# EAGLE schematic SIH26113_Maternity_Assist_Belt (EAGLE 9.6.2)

## Sheet 1 of 7: SHEET 1/7 - POWER ENTRY, CHARGING AND 3V3 REGULATION
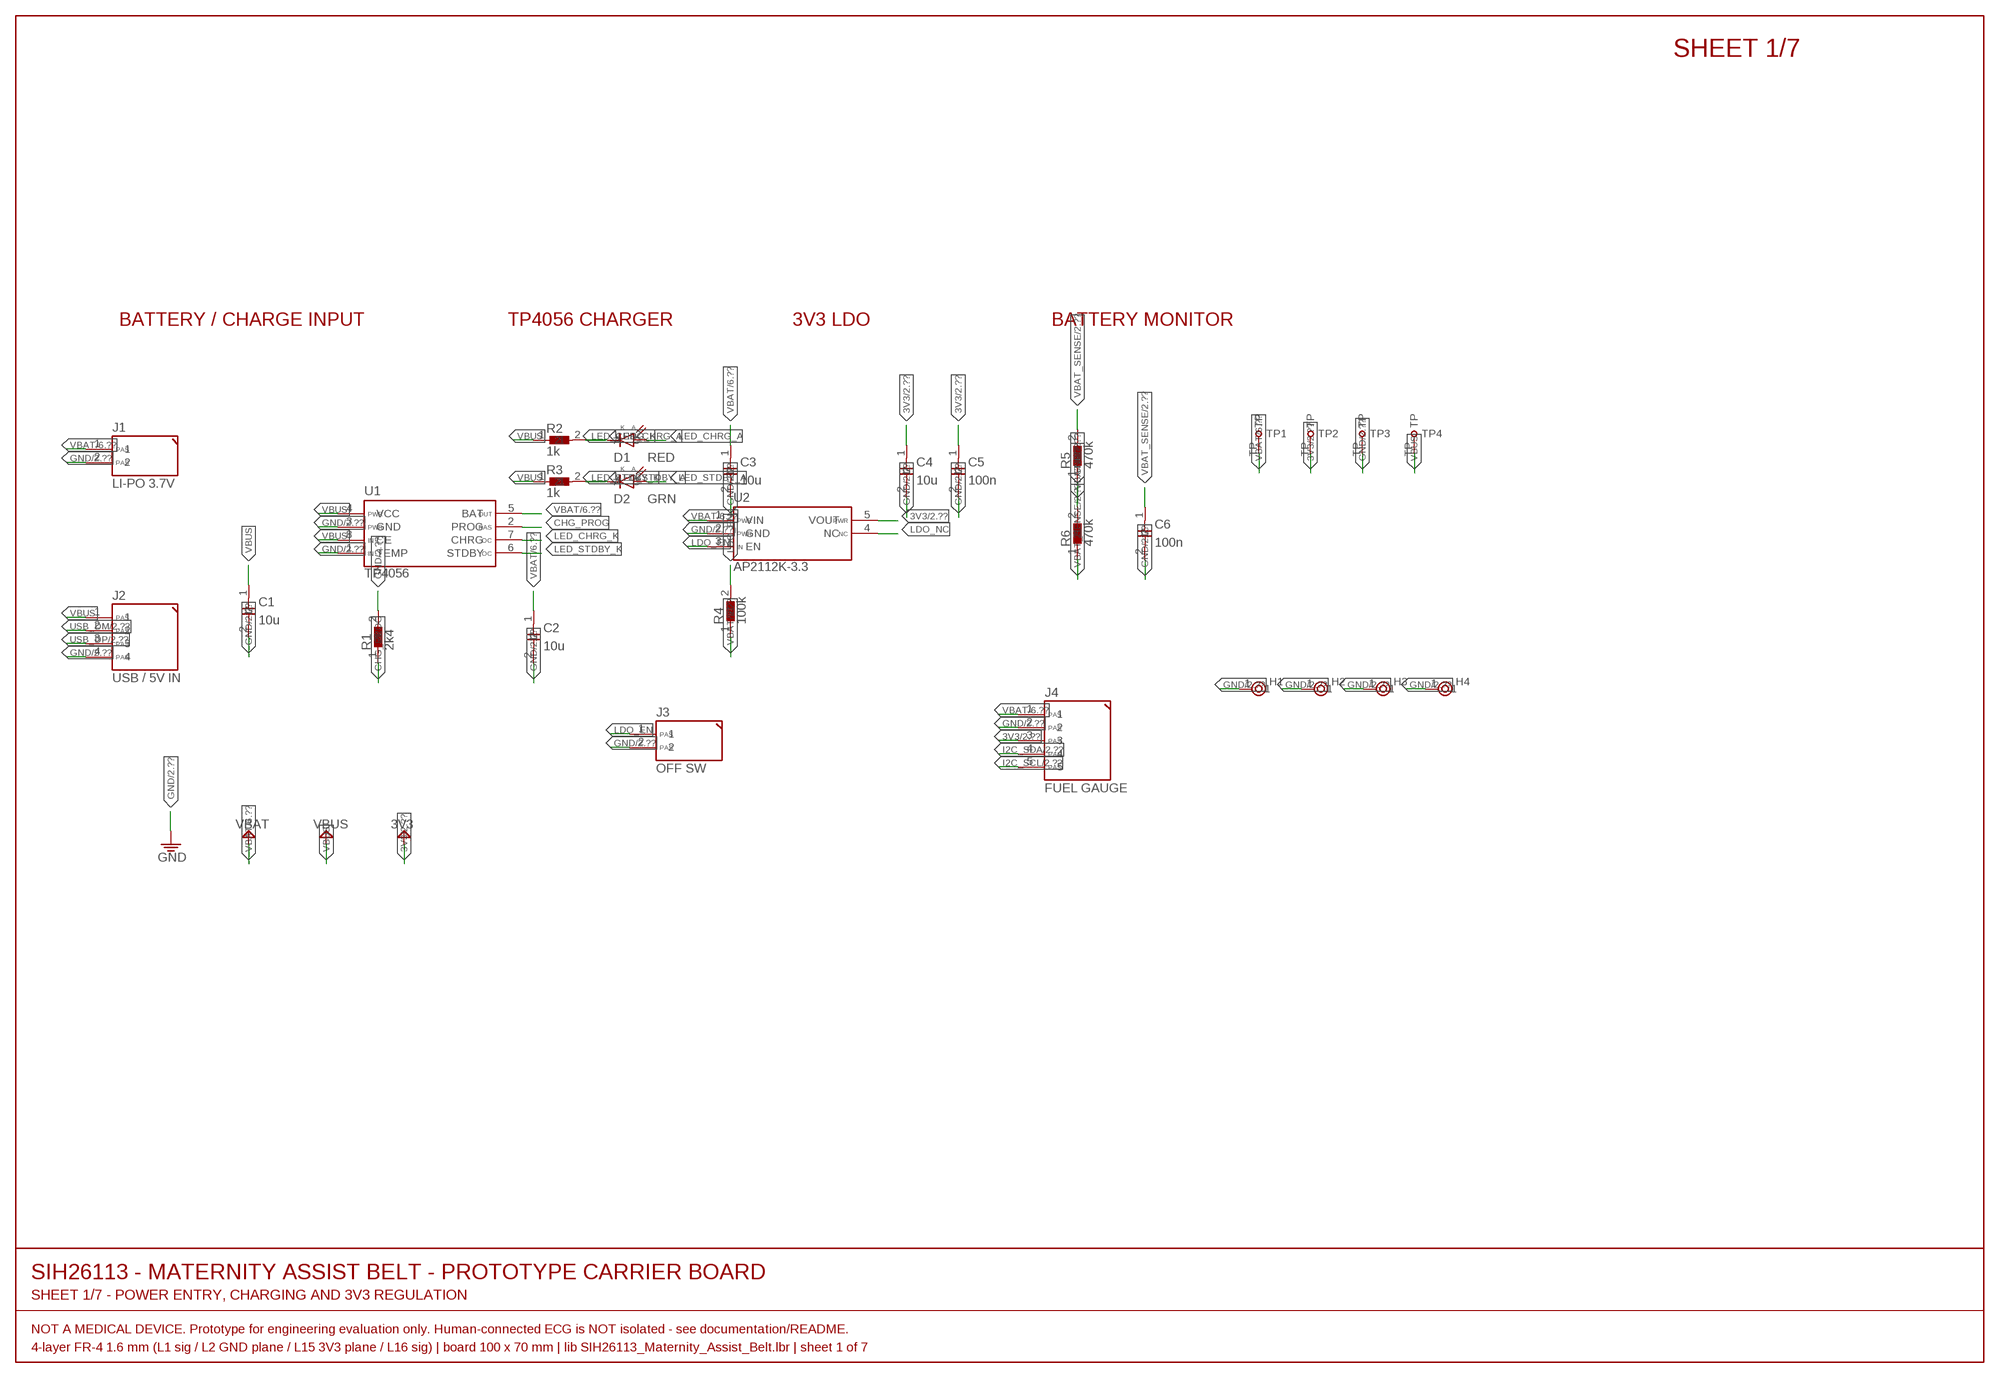
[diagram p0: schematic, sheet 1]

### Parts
C1  10u  C-0805  [C0805]
C2  10u  C-0805  [C0805]
C3  10u  C-0805  [C0805]
C4  10u  C-0805  [C0805]
C5  100n  C-0805  [C0805]
C6  100n  C-0805  [C0805]
D1  RED  LED-0805  [LED0805]
D2  GRN  LED-0805  [LED0805]
H1  M2  MOUNTHOLE-M2  [MOUNT-M2]
H2  M2  MOUNTHOLE-M2  [MOUNT-M2]
H3  M2  MOUNTHOLE-M2  [MOUNT-M2]
H4  M2  MOUNTHOLE-M2  [MOUNT-M2]
J1  LI-PO 3.7V  JST-PH-2  [JST-PH-2]
J2  USB / 5V IN  HDR-1X4  [HDR-1X4]
J3  OFF SW  HDR-1X2  [HDR-1X2]
J4  FUEL GAUGE  HDR-1X5  [HDR-1X5]
R1  2k4  R-0805  [R0805]
R2  1k  R-0805  [R0805]
R3  1k  R-0805  [R0805]
R4  100k  R-0805  [R0805]
R5  470k  R-0805  [R0805]
R6  470k  R-0805  [R0805]
TP1  VBAT  TESTPOINT  [TESTPOINT-1.5]
TP2  3V3  TESTPOINT  [TESTPOINT-1.5]
TP3  GND  TESTPOINT  [TESTPOINT-1.5]
TP4  VBUS  TESTPOINT  [TESTPOINT-1.5]
U1  TP4056  [SOIC-8-N]
U2  AP2112K-3.3  [SOT-23-5]

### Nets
3V3 [power]: C4.1 C5.1 J4.3 TP2.TP U2.5(VOUT) ; also sheet 2,3,4,5,6,7
CHG_PROG: R1.1 U1.2(PROG)
GND [power]: C1.2 C2.2 C3.2 C4.2 C5.2 C6.2 H1.1 H2.1 H3.1 H4.1 J1.2 J2.4 J3.2 J4.2 R1.2 R6.2 TP3.TP U1.1(TEMP) U1.3(GND) U2.2(GND) ; also sheet 2,3,4,5,6,7
I2C_SCL: J4.5 ; also sheet 2,3,7
I2C_SDA: J4.4 ; also sheet 2,3,7
LDO_EN: J3.1 R4.2 U2.3(EN)
LDO_NC: U2.4(NC)
LED_CHRG_A: D1.2(A) R2.2
LED_CHRG_K: D1.1(C) U1.7(CHRG)
LED_STDBY_A: D2.2(A) R3.2
LED_STDBY_K: D2.1(C) U1.6(STDBY)
USB_DM: J2.2 ; also sheet 2
USB_DP: J2.3 ; also sheet 2
VBAT [power]: C2.1 C3.1 J1.1 J4.1 R4.1 R5.1 TP1.TP U1.5(BAT) U2.1(VIN) ; also sheet 6
VBAT_SENSE: C6.1 R5.2 R6.1 ; also sheet 2
VBUS [power]: C1.1 J2.1 R2.1 R3.1 TP4.TP U1.4(VCC) U1.8(CE)

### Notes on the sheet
- SHEET 1/7
- BATTERY / CHARGE INPUT | TP4056 CHARGER | 3V3 LDO | BATTERY MONITOR
- SIH26113 - MATERNITY ASSIST BELT - PROTOTYPE CARRIER BOARD
- SHEET 1/7 - POWER ENTRY, CHARGING AND 3V3 REGULATION
- NOT A MEDICAL DEVICE. Prototype for engineering evaluation only. Human-connected ECG is NOT isolated - see documentation/README.
- 4-layer FR-4 1.6 mm (L1 sig / L2 GND plane / L15 3V3 plane / L16 sig) | board 100 x 70 mm | lib SIH26113_Maternity_Assist_Belt.lbr | sheet 1 of 7

## Sheet 2 of 7: SHEET 2/7 - ESP32-S3 CENTRAL MCU, RESET/BOOT, PROGRAMMING, INDICATORS
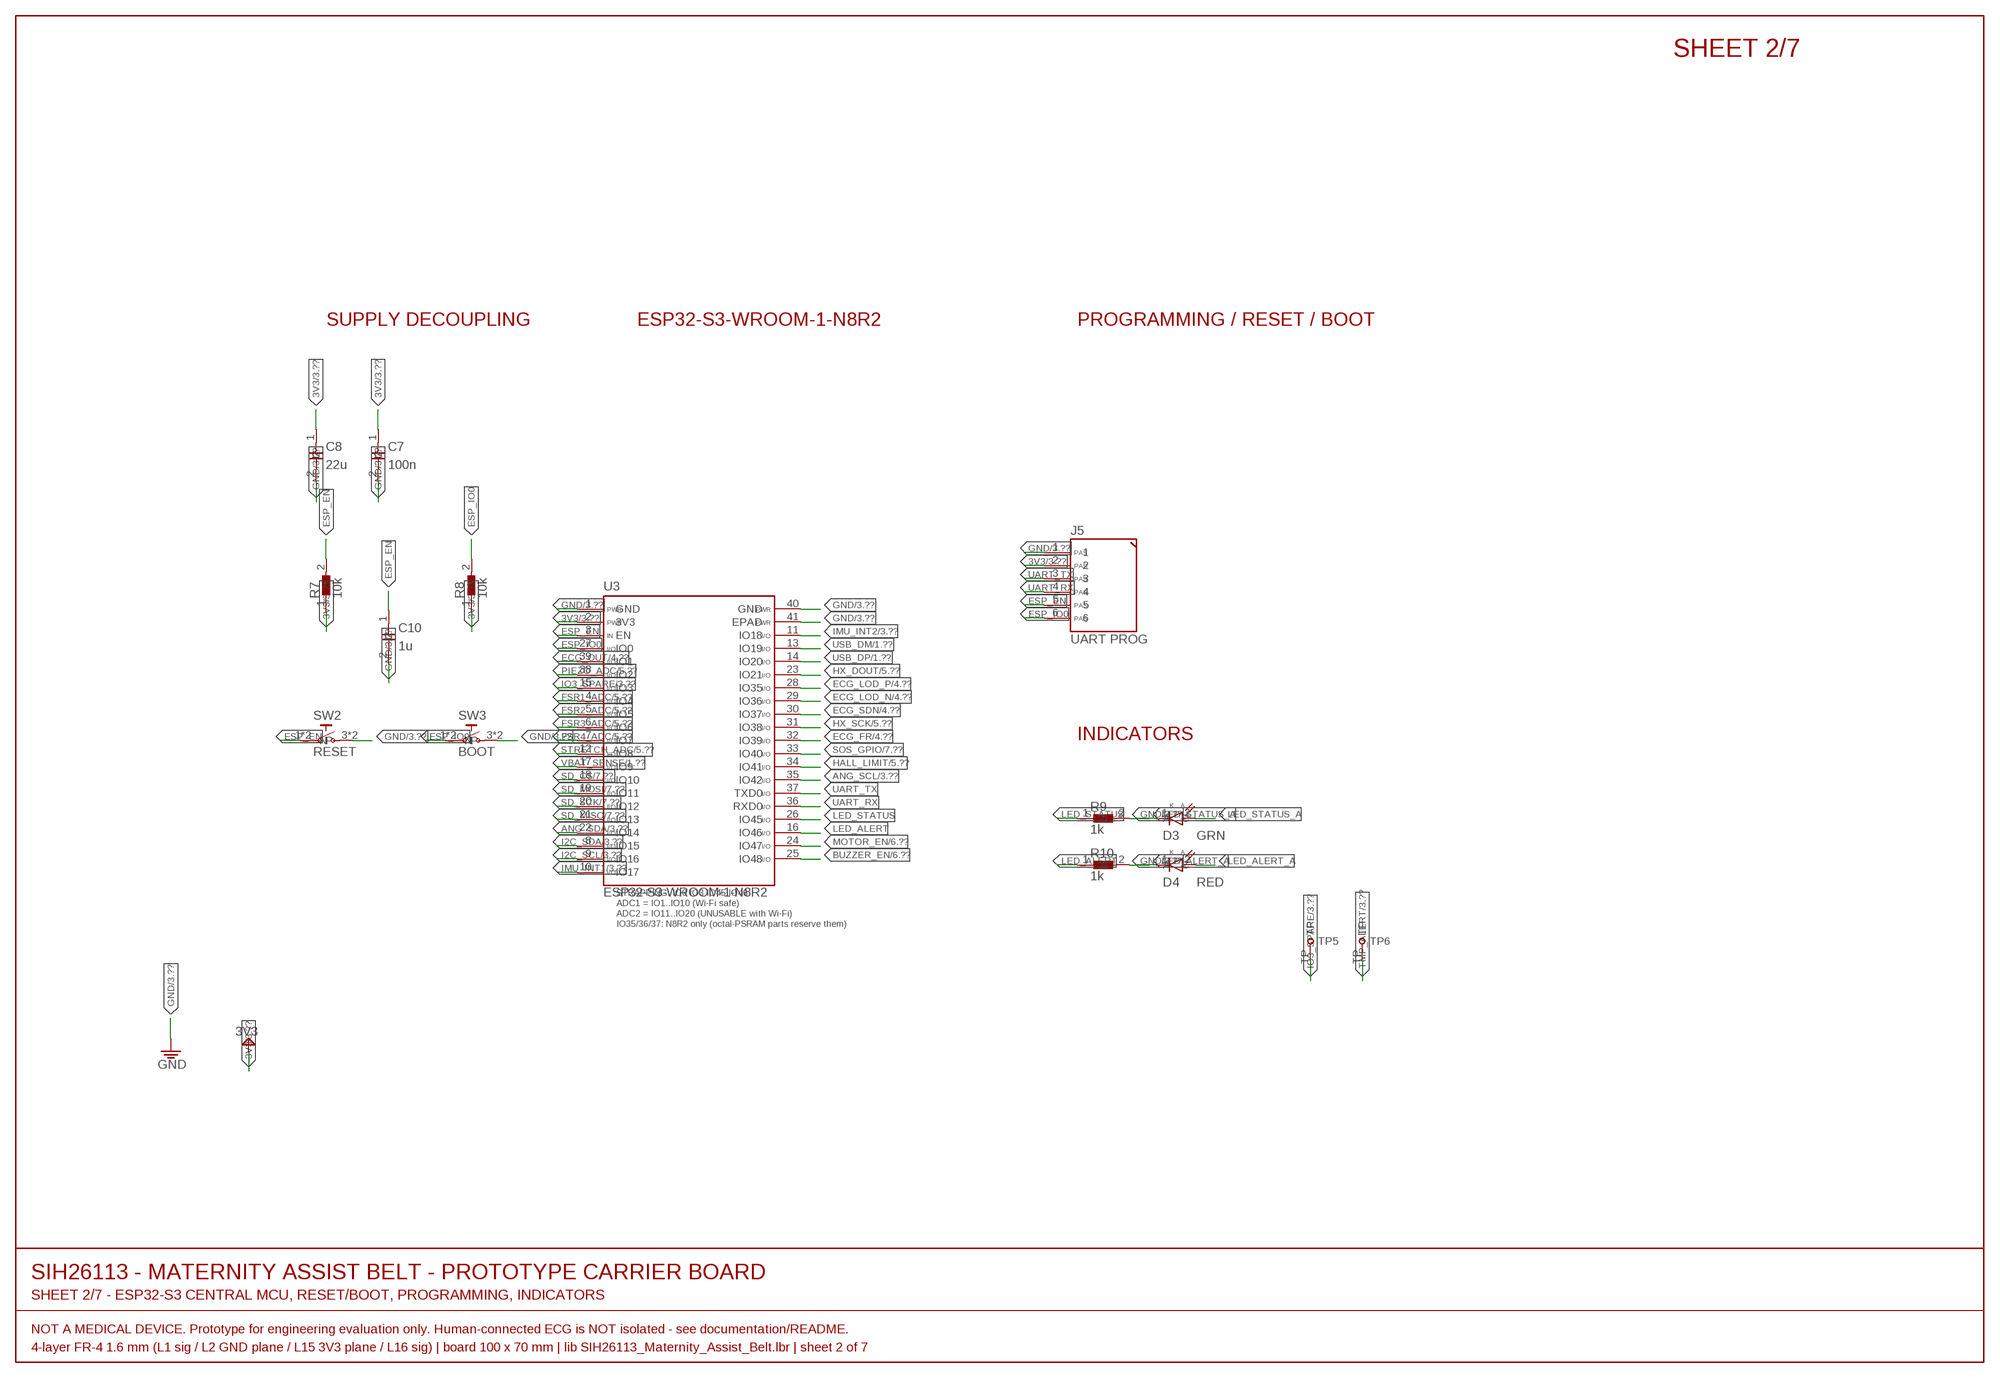
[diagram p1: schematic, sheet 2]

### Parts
C7  100n  C-0805  [C0805]
C8  22u  C-0805  [C0805]
C10  1u  C-0805  [C0805]
D3  GRN  LED-0805  [LED0805]
D4  RED  LED-0805  [LED0805]
J5  UART PROG  HDR-1X6  [HDR-1X6]
R7  10k  R-0805  [R0805]
R8  10k  R-0805  [R0805]
R9  1k  R-0805  [R0805]
R10  1k  R-0805  [R0805]
SW2  RESET  SW-TACT-6MM  [TACT-6X6-THT]
SW3  BOOT  SW-TACT-6MM  [TACT-6X6-THT]
TP5  IO3  TESTPOINT  [TESTPOINT-1.5]
TP6  TMP_ALERT  TESTPOINT  [TESTPOINT-1.5]
U3  ESP32-S3-WROOM-1-N8R2  ESP32-S3-WROOM-1  [ESP32-S3-WROOM-1]

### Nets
3V3 [power]: C7.1 C8.1 J5.2 R7.1 R8.1 U3.2(3V3) ; also sheet 1,3,4,5,6,7
ANG_SCL: U3.35(IO42) ; also sheet 3
ANG_SDA: U3.22(IO14) ; also sheet 3
BUZZER_EN: U3.25(IO48) ; also sheet 6
ECG_FR: U3.32(IO39) ; also sheet 4
ECG_LOD_N: U3.29(IO36) ; also sheet 4
ECG_LOD_P: U3.28(IO35) ; also sheet 4
ECG_OUT [analog_ecg]: U3.39(IO1) ; also sheet 4
ECG_SDN: U3.30(IO37) ; also sheet 4
ESP_EN: C10.1 J5.5 R7.2 SW2.1(P) SW2.2(P) U3.3(EN)
ESP_IO0: J5.6 R8.2 SW3.1(P) SW3.2(P) U3.27(IO0)
FSR1_ADC: U3.4(IO4) ; also sheet 5
FSR2_ADC: U3.5(IO5) ; also sheet 5
FSR3_ADC: U3.6(IO6) ; also sheet 5
FSR4_ADC: U3.7(IO7) ; also sheet 5
GND [power]: C7.2 C8.2 C10.2 D3.1(C) D4.1(C) J5.1 SW2.3(N) SW2.4(N) SW3.3(N) SW3.4(N) U3.1(GND) U3.40(GND) U3.41(EPAD) ; also sheet 1,3,4,5,6,7
HALL_LIMIT: U3.34(IO41) ; also sheet 5
HX_DOUT: U3.23(IO21) ; also sheet 5
HX_SCK: U3.31(IO38) ; also sheet 5
I2C_SCL: U3.9(IO16) ; also sheet 1,3,7
I2C_SDA: U3.8(IO15) ; also sheet 1,3,7
IMU_INT1: U3.10(IO17) ; also sheet 3
IMU_INT2: U3.11(IO18) ; also sheet 3
IO3_SPARE: TP5.TP U3.15(IO3) ; also sheet 3
LED_ALERT: R10.1 U3.16(IO46)
LED_ALERT_A: D4.2(A) R10.2
LED_STATUS: R9.1 U3.26(IO45)
LED_STATUS_A: D3.2(A) R9.2
MOTOR_EN: U3.24(IO47) ; also sheet 6
PIEZO_ADC: U3.38(IO2) ; also sheet 5
SD_CS: U3.18(IO10) ; also sheet 7
SD_MISO: U3.21(IO13) ; also sheet 7
SD_MOSI: U3.19(IO11) ; also sheet 7
SD_SCK: U3.20(IO12) ; also sheet 7
SOS_GPIO: U3.33(IO40) ; also sheet 7
STRETCH_ADC: U3.12(IO8) ; also sheet 5
TMP_ALERT: TP6.TP ; also sheet 3
UART_RX: J5.4 U3.36(RXD0)
UART_TX: J5.3 U3.37(TXD0)
USB_DM: U3.13(IO19) ; also sheet 1
USB_DP: U3.14(IO20) ; also sheet 1
VBAT_SENSE: U3.17(IO9) ; also sheet 1

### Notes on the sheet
- SHEET 2/7
- SUPPLY DECOUPLING | ESP32-S3-WROOM-1-N8R2 | PROGRAMMING / RESET / BOOT
- INDICATORS
- SIH26113 - MATERNITY ASSIST BELT - PROTOTYPE CARRIER BOARD
- SHEET 2/7 - ESP32-S3 CENTRAL MCU, RESET/BOOT, PROGRAMMING, INDICATORS
- NOT A MEDICAL DEVICE. Prototype for engineering evaluation only. Human-connected ECG is NOT isolated - see documentation/README.
- 4-layer FR-4 1.6 mm (L1 sig / L2 GND plane / L15 3V3 plane / L16 sig) | board 100 x 70 mm | lib SIH26113_Maternity_Assist_Belt.lbr | sheet 2 of 7

## Sheet 3 of 7: SHEET 3/7 - I2C SENSORS (TMP117, LSM6DSOX, AS5600) - TWO BUSSES
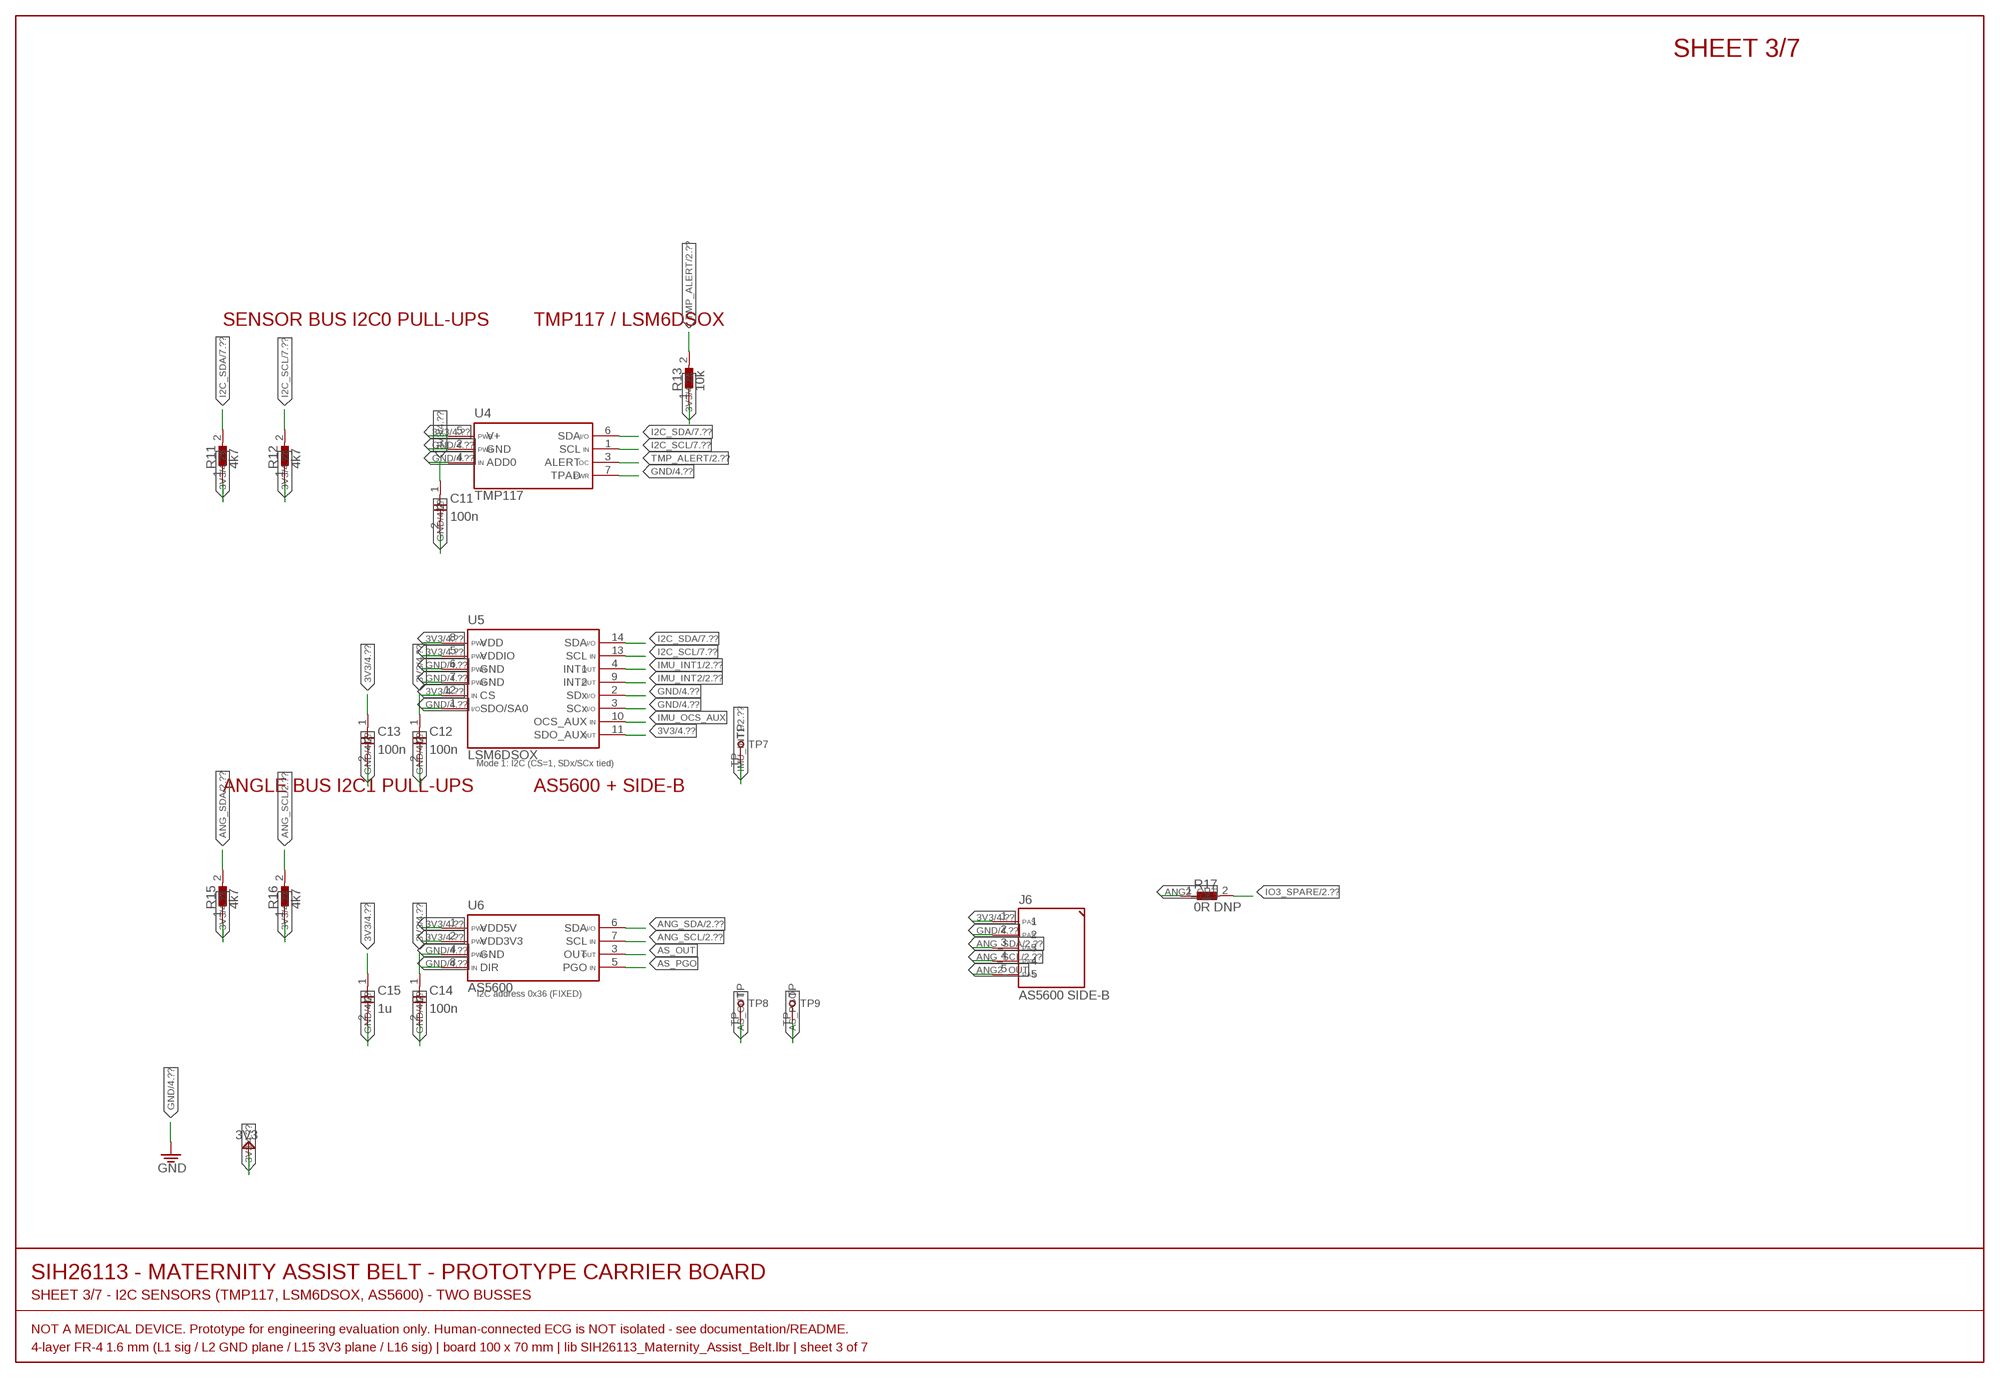
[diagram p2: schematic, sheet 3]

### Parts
C11  100n  C-0805  [C0805]
C12  100n  C-0805  [C0805]
C13  100n  C-0805  [C0805]
C14  100n  C-0805  [C0805]
C15  1u  C-0805  [C0805]
J6  AS5600 SIDE-B  HDR-1X5  [HDR-1X5]
R11  4k7  R-0805  [R0805]
R12  4k7  R-0805  [R0805]
R13  10k  R-0805  [R0805]
R15  4k7  R-0805  [R0805]
R16  4k7  R-0805  [R0805]
R17  0R DNP  R-0805  [R0805]
TP7  IMU_INT1  TESTPOINT  [TESTPOINT-1.5]
TP8  AS_OUT  TESTPOINT  [TESTPOINT-1.5]
TP9  AS_PGO  TESTPOINT  [TESTPOINT-1.5]
U4  TMP117  [WSON-6-DRV0006B]
U5  LSM6DSOX  [LGA-14L-2.5X3.0]
U6  AS5600  [SOIC-8-N]

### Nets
3V3 [power]: C11.1 C12.1 C13.1 C14.1 C15.1 J6.1 R11.1 R12.1 R13.1 R15.1 R16.1 U4.5(V+) U5.5(VDDIO) U5.8(VDD) U5.11(SDO_AUX) U5.12(CS) U6.1(VDD5V) U6.2(VDD3V3) ; also sheet 1,2,4,5,6,7
ANG2_OUT: J6.5 R17.1
ANG_SCL: J6.4 R16.2 U6.7(SCL) ; also sheet 2
ANG_SDA: J6.3 R15.2 U6.6(SDA) ; also sheet 2
AS_OUT: TP8.TP U6.3(OUT)
AS_PGO: TP9.TP U6.5(PGO)
GND [power]: C11.2 C12.2 C13.2 C14.2 C15.2 J6.2 U4.2(GND) U4.4(ADD0) U4.7(TPAD) U5.1(SDO/SA0) U5.2(SDx) U5.3(SCx) U5.6(GND) U5.7(GND) U6.4(GND) U6.8(DIR) ; also sheet 1,2,4,5,6,7
I2C_SCL: R12.2 U4.1(SCL) U5.13(SCL) ; also sheet 1,2,7
I2C_SDA: R11.2 U4.6(SDA) U5.14(SDA) ; also sheet 1,2,7
IMU_INT1: TP7.TP U5.4(INT1) ; also sheet 2
IMU_INT2: U5.9(INT2) ; also sheet 2
IMU_OCS_AUX: U5.10(OCS_AUX)
IO3_SPARE: R17.2 ; also sheet 2
TMP_ALERT: R13.2 U4.3(ALERT) ; also sheet 2

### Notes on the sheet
- SHEET 3/7
- SENSOR BUS I2C0 PULL-UPS | TMP117 / LSM6DSOX
- ANGLE BUS I2C1 PULL-UPS | AS5600 + SIDE-B
- SIH26113 - MATERNITY ASSIST BELT - PROTOTYPE CARRIER BOARD
- SHEET 3/7 - I2C SENSORS (TMP117, LSM6DSOX, AS5600) - TWO BUSSES
- NOT A MEDICAL DEVICE. Prototype for engineering evaluation only. Human-connected ECG is NOT isolated - see documentation/README.
- 4-layer FR-4 1.6 mm (L1 sig / L2 GND plane / L15 3V3 plane / L16 sig) | board 100 x 70 mm | lib SIH26113_Maternity_Assist_Belt.lbr | sheet 3 of 7

## Sheet 4 of 7: SHEET 4/7 - ECG ANALOG FRONT END (AD8232)
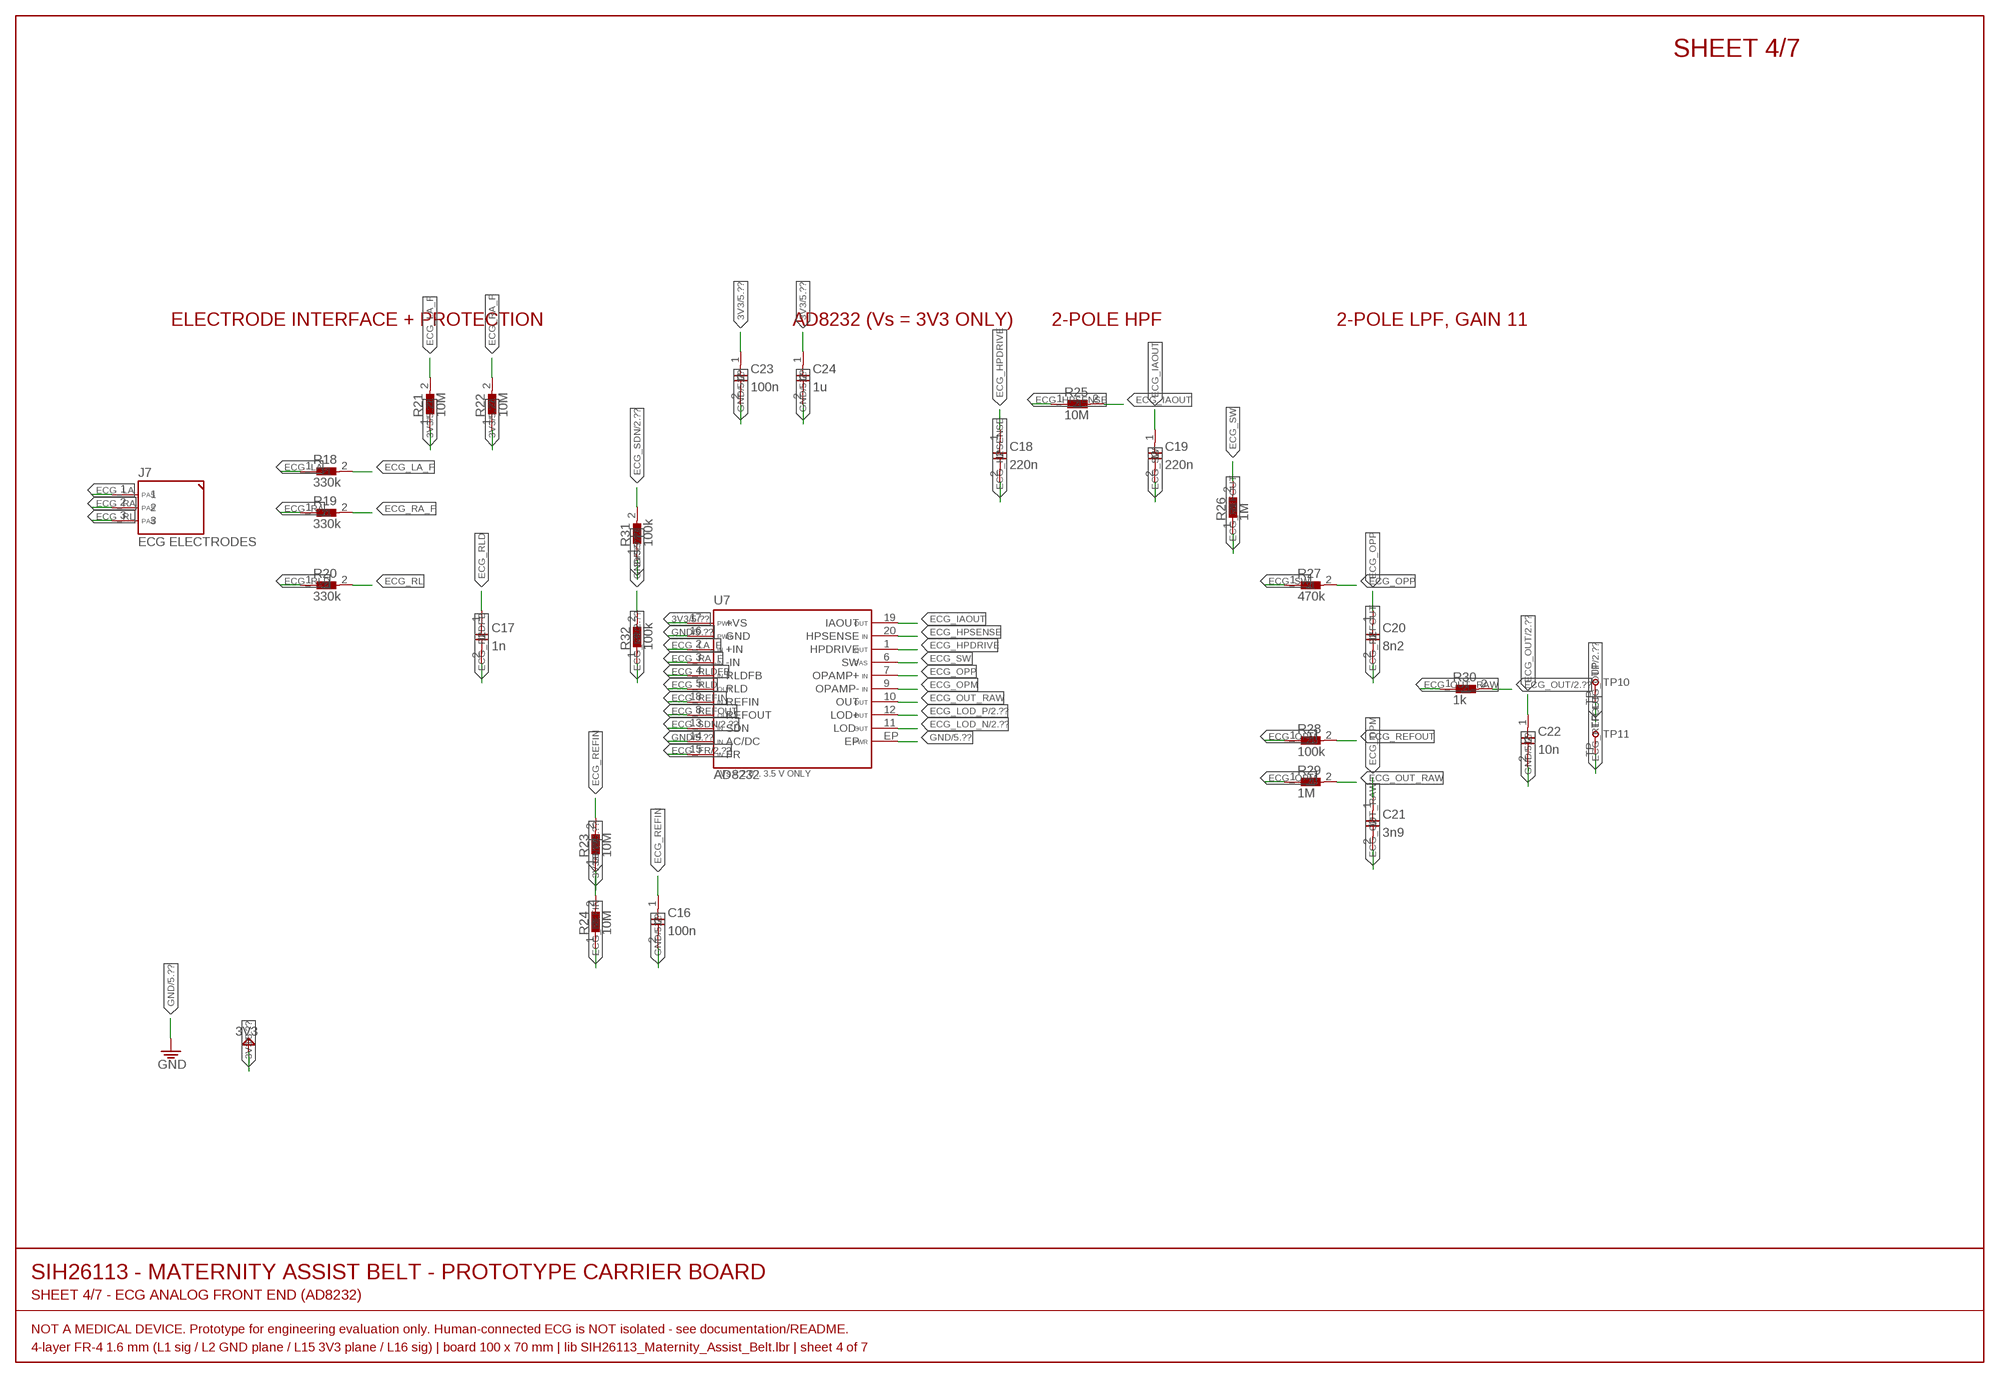
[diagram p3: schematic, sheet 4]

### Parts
C16  100n  C-0805  [C0805]
C17  1n  C-0805  [C0805]
C18  220n  C-0805  [C0805]
C19  220n  C-0805  [C0805]
C20  8n2  C-0805  [C0805]
C21  3n9  C-0805  [C0805]
C22  10n  C-0805  [C0805]
C23  100n  C-0805  [C0805]
C24  1u  C-0805  [C0805]
J7  ECG ELECTRODES  HDR-1X3  [HDR-1X3]
R18  330k  R-0805  [R0805]
R19  330k  R-0805  [R0805]
R20  330k  R-0805  [R0805]
R21  10M  R-0805  [R0805]
R22  10M  R-0805  [R0805]
R23  10M  R-0805  [R0805]
R24  10M  R-0805  [R0805]
R25  10M  R-0805  [R0805]
R26  1M  R-0805  [R0805]
R27  470k  R-0805  [R0805]
R28  100k  R-0805  [R0805]
R29  1M  R-0805  [R0805]
R30  1k  R-0805  [R0805]
R31  100k  R-0805  [R0805]
R32  100k  R-0805  [R0805]
TP10  ECG_OUT  TESTPOINT  [TESTPOINT-1.5]
TP11  ECG_REF  TESTPOINT  [TESTPOINT-1.5]
U7  AD8232  [LFCSP-20-4X4-P050]

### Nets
3V3 [power]: C23.1 C24.1 R21.1 R22.1 R23.1 R31.1 U7.17(+VS) ; also sheet 1,2,3,5,6,7
ECG_FR: R32.1 U7.15(FR) ; also sheet 2
ECG_HPDRIVE: C18.1 U7.1(HPDRIVE)
ECG_HPSENSE [analog_ecg]: C18.2 R25.1 U7.20(HPSENSE)
ECG_IAOUT [analog_ecg]: C19.1 R25.2 U7.19(IAOUT)
ECG_LA [analog_ecg]: J7.1 R18.1
ECG_LA_F [analog_ecg]: R18.2 R21.2 U7.2(+IN)
ECG_LOD_N: U7.11(LOD-) ; also sheet 2
ECG_LOD_P: U7.12(LOD+) ; also sheet 2
ECG_OPM [analog_ecg]: C21.1 R28.1 R29.1 U7.9(OPAMP-)
ECG_OPP [analog_ecg]: C20.1 R27.2 U7.7(OPAMP+)
ECG_OUT [analog_ecg]: C22.1 R30.2 TP10.TP ; also sheet 2
ECG_OUT_RAW [analog_ecg]: C21.2 R29.2 R30.1 U7.10(OUT)
ECG_RA [analog_ecg]: J7.2 R19.1
ECG_RA_F [analog_ecg]: R19.2 R22.2 U7.3(-IN)
ECG_REFIN [analog_ecg]: C16.1 R23.2 R24.1 U7.18(REFIN)
ECG_REFOUT [analog_ecg]: C20.2 R26.1 R28.2 TP11.TP U7.8(REFOUT)
ECG_RL [analog_ecg]: J7.3 R20.2
ECG_RLD [analog_ecg]: C17.1 R20.1 U7.5(RLD)
ECG_RLDFB: C17.2 U7.4(RLDFB)
ECG_SDN: R31.2 U7.13(SDN) ; also sheet 2
ECG_SW [analog_ecg]: C19.2 R26.2 R27.1 U7.6(SW)
GND [power]: C16.2 C22.2 C23.2 C24.2 R24.2 R32.2 U7.14(AC/DC) U7.16(GND) U7.EP ; also sheet 1,2,3,5,6,7

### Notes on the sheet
- SHEET 4/7
- ELECTRODE INTERFACE + PROTECTION | AD8232 (Vs = 3V3 ONLY) | 2-POLE HPF | 2-POLE LPF, GAIN 11
- SIH26113 - MATERNITY ASSIST BELT - PROTOTYPE CARRIER BOARD
- SHEET 4/7 - ECG ANALOG FRONT END (AD8232)
- NOT A MEDICAL DEVICE. Prototype for engineering evaluation only. Human-connected ECG is NOT isolated - see documentation/README.
- 4-layer FR-4 1.6 mm (L1 sig / L2 GND plane / L15 3V3 plane / L16 sig) | board 100 x 70 mm | lib SIH26113_Maternity_Assist_Belt.lbr | sheet 4 of 7

## Sheet 5 of 7: SHEET 5/7 - MECHANICAL SENSING (LOAD CELL, FSR, STRETCH, PIEZO, HALL)
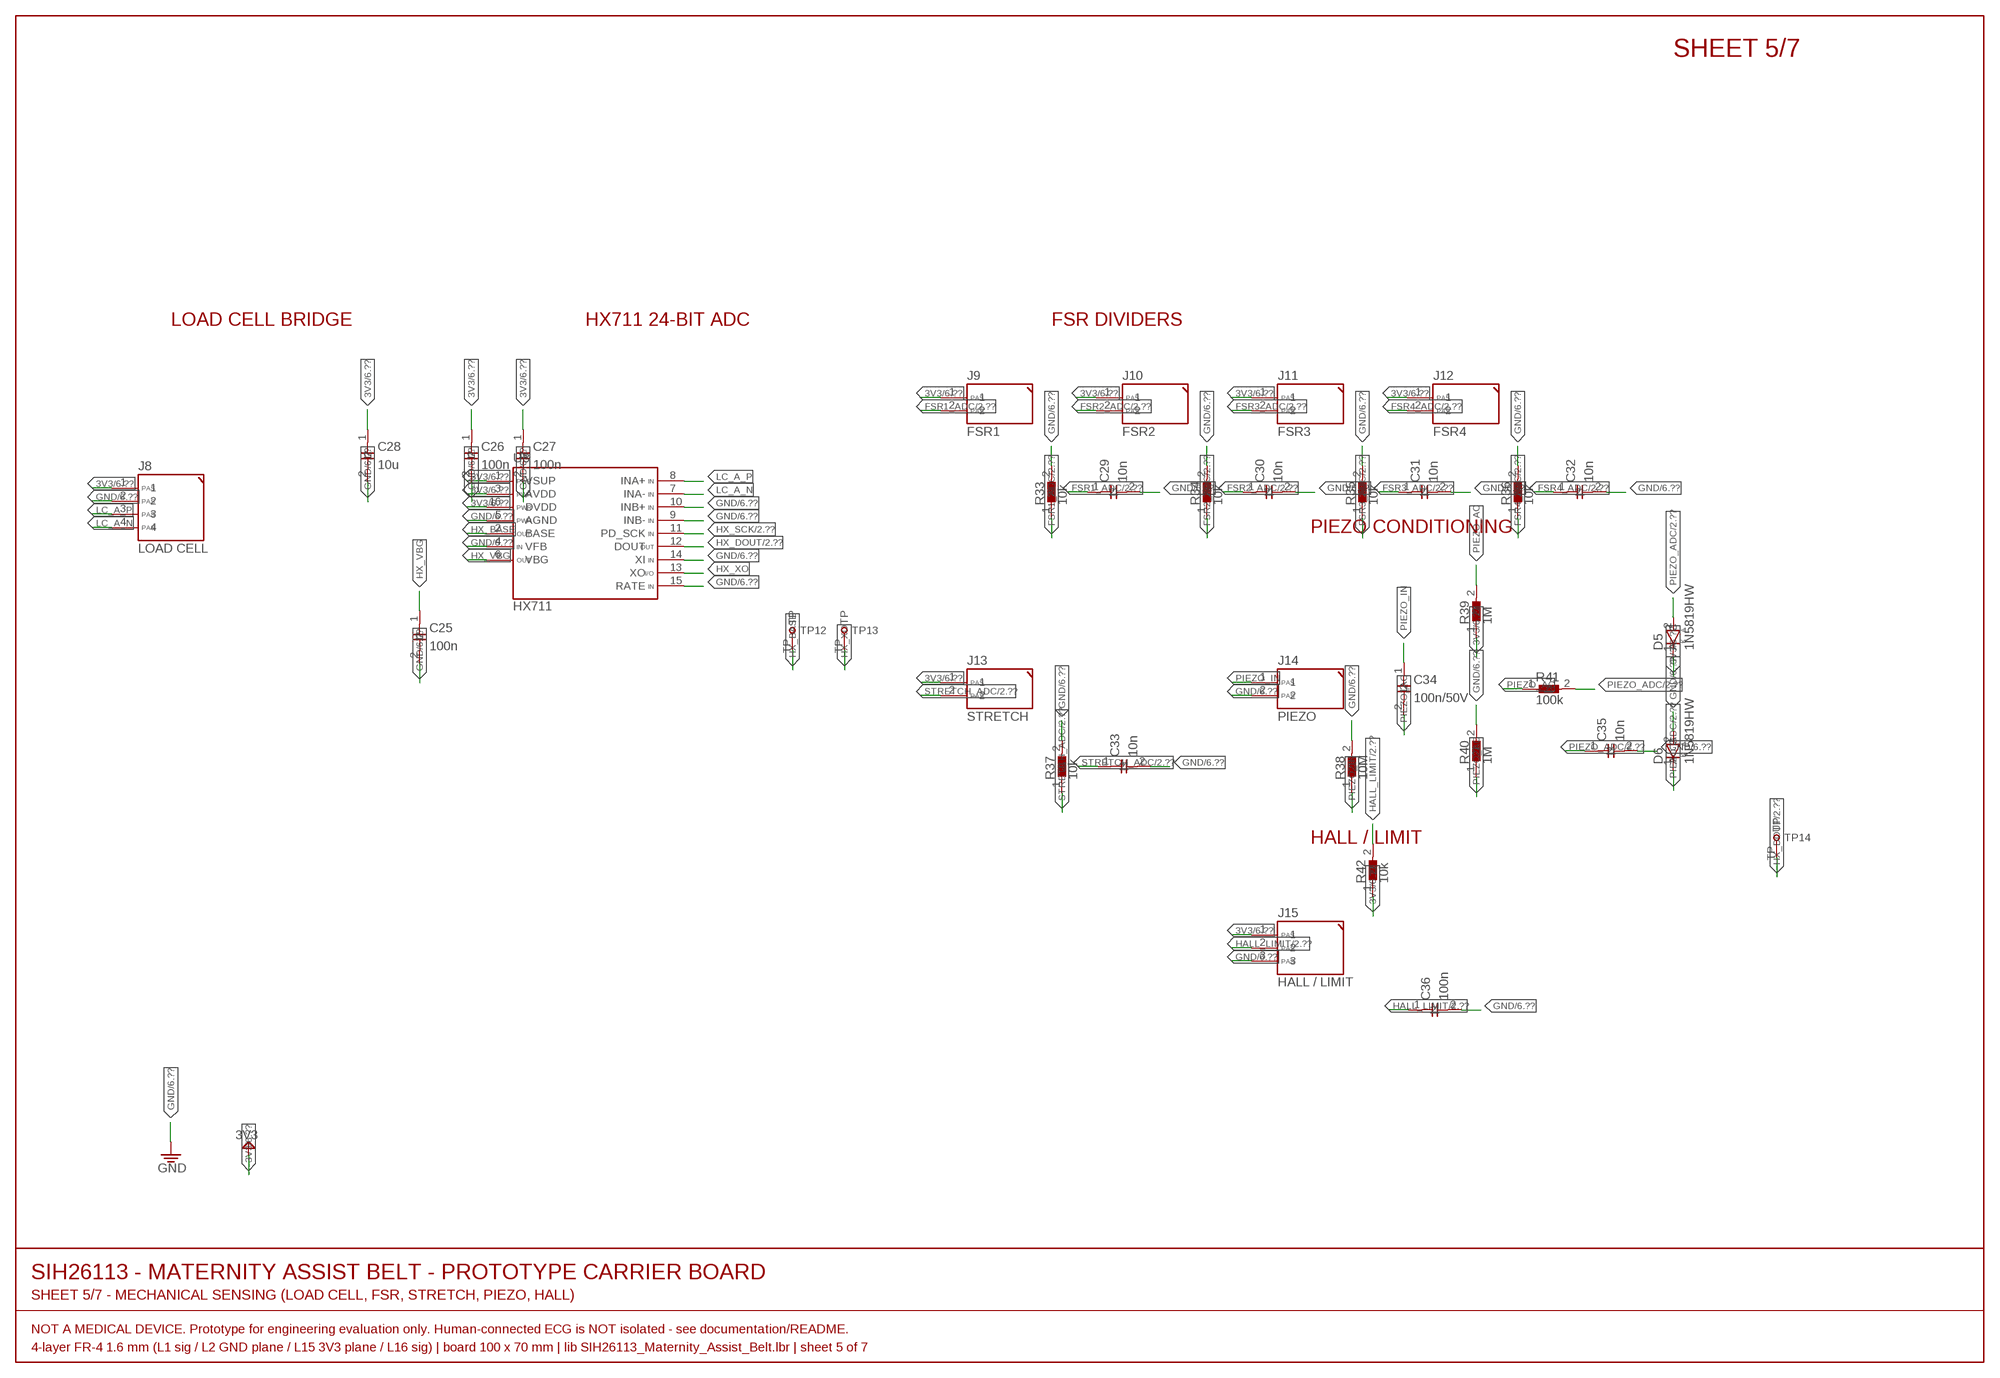
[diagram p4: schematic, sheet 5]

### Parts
C25  100n  C-0805  [C0805]
C26  100n  C-0805  [C0805]
C27  100n  C-0805  [C0805]
C28  10u  C-0805  [C0805]
C29  10n  C-0805  [C0805]
C30  10n  C-0805  [C0805]
C31  10n  C-0805  [C0805]
C32  10n  C-0805  [C0805]
C33  10n  C-0805  [C0805]
C34  100n/50V  C-0805  [C0805]
C35  10n  C-0805  [C0805]
C36  100n  C-0805  [C0805]
D5  1N5819HW  DIODE-SOD123  [SOD-123]
D6  1N5819HW  DIODE-SOD123  [SOD-123]
J8  LOAD CELL  JST-PH-4  [JST-PH-4]
J9  FSR1  HDR-1X2  [HDR-1X2]
J10  FSR2  HDR-1X2  [HDR-1X2]
J11  FSR3  HDR-1X2  [HDR-1X2]
J12  FSR4  HDR-1X2  [HDR-1X2]
J13  STRETCH  HDR-1X2  [HDR-1X2]
J14  PIEZO  HDR-1X2  [HDR-1X2]
J15  HALL / LIMIT  HDR-1X3  [HDR-1X3]
R33  10k  R-0805  [R0805]
R34  10k  R-0805  [R0805]
R35  10k  R-0805  [R0805]
R36  10k  R-0805  [R0805]
R37  10k  R-0805  [R0805]
R38  10M  R-0805  [R0805]
R39  1M  R-0805  [R0805]
R40  1M  R-0805  [R0805]
R41  100k  R-0805  [R0805]
R42  10k  R-0805  [R0805]
TP12  HX_BASE  TESTPOINT  [TESTPOINT-1.5]
TP13  HX_XO  TESTPOINT  [TESTPOINT-1.5]
TP14  HX_DOUT  TESTPOINT  [TESTPOINT-1.5]
U8  HX711  [SOP-16-N]

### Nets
3V3 [power]: C26.1 C27.1 C28.1 D5.1(C) J8.1 J9.1 J10.1 J11.1 J12.1 J13.1 J15.1 R39.1 R42.1 U8.1(VSUP) U8.3(AVDD) U8.16(DVDD) ; also sheet 1,2,3,4,6,7
FSR1_ADC: C29.1 J9.2 R33.1 ; also sheet 2
FSR2_ADC: C30.1 J10.2 R34.1 ; also sheet 2
FSR3_ADC: C31.1 J11.2 R35.1 ; also sheet 2
FSR4_ADC: C32.1 J12.2 R36.1 ; also sheet 2
GND [power]: C25.2 C26.2 C27.2 C28.2 C29.2 C30.2 C31.2 C32.2 C33.2 C35.2 C36.2 D6.2(A) J8.2 J14.2 J15.3 R33.2 R34.2 R35.2 R36.2 R37.2 R38.2 R40.2 U8.4(VFB) U8.5(AGND) U8.9(INB-) U8.10(INB+) U8.14(XI) U8.15(RATE) ; also sheet 1,2,3,4,6,7
HALL_LIMIT: C36.1 J15.2 R42.2 ; also sheet 2
HX_BASE: TP12.TP U8.2(BASE)
HX_DOUT: TP14.TP U8.12(DOUT) ; also sheet 2
HX_SCK: U8.11(PD_SCK) ; also sheet 2
HX_VBG: C25.1 U8.6(VBG)
HX_XO: TP13.TP U8.13(XO)
LC_A_N: J8.4 U8.7(INA-)
LC_A_P: J8.3 U8.8(INA+)
PIEZO_AC: C34.2 R39.2 R40.1 R41.1
PIEZO_ADC: C35.1 D5.2(A) D6.1(C) R41.2 ; also sheet 2
PIEZO_IN: C34.1 J14.1 R38.1
STRETCH_ADC: C33.1 J13.2 R37.1 ; also sheet 2

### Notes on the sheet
- SHEET 5/7
- LOAD CELL BRIDGE | HX711 24-BIT ADC | FSR DIVIDERS
- PIEZO CONDITIONING
- HALL / LIMIT
- SIH26113 - MATERNITY ASSIST BELT - PROTOTYPE CARRIER BOARD
- SHEET 5/7 - MECHANICAL SENSING (LOAD CELL, FSR, STRETCH, PIEZO, HALL)
- NOT A MEDICAL DEVICE. Prototype for engineering evaluation only. Human-connected ECG is NOT isolated - see documentation/README.
- 4-layer FR-4 1.6 mm (L1 sig / L2 GND plane / L15 3V3 plane / L16 sig) | board 100 x 70 mm | lib SIH26113_Maternity_Assist_Belt.lbr | sheet 5 of 7

## Sheet 6 of 7: SHEET 6/7 - FET-DRIVEN ALERTS (VIBRATION MOTOR, BUZZER)
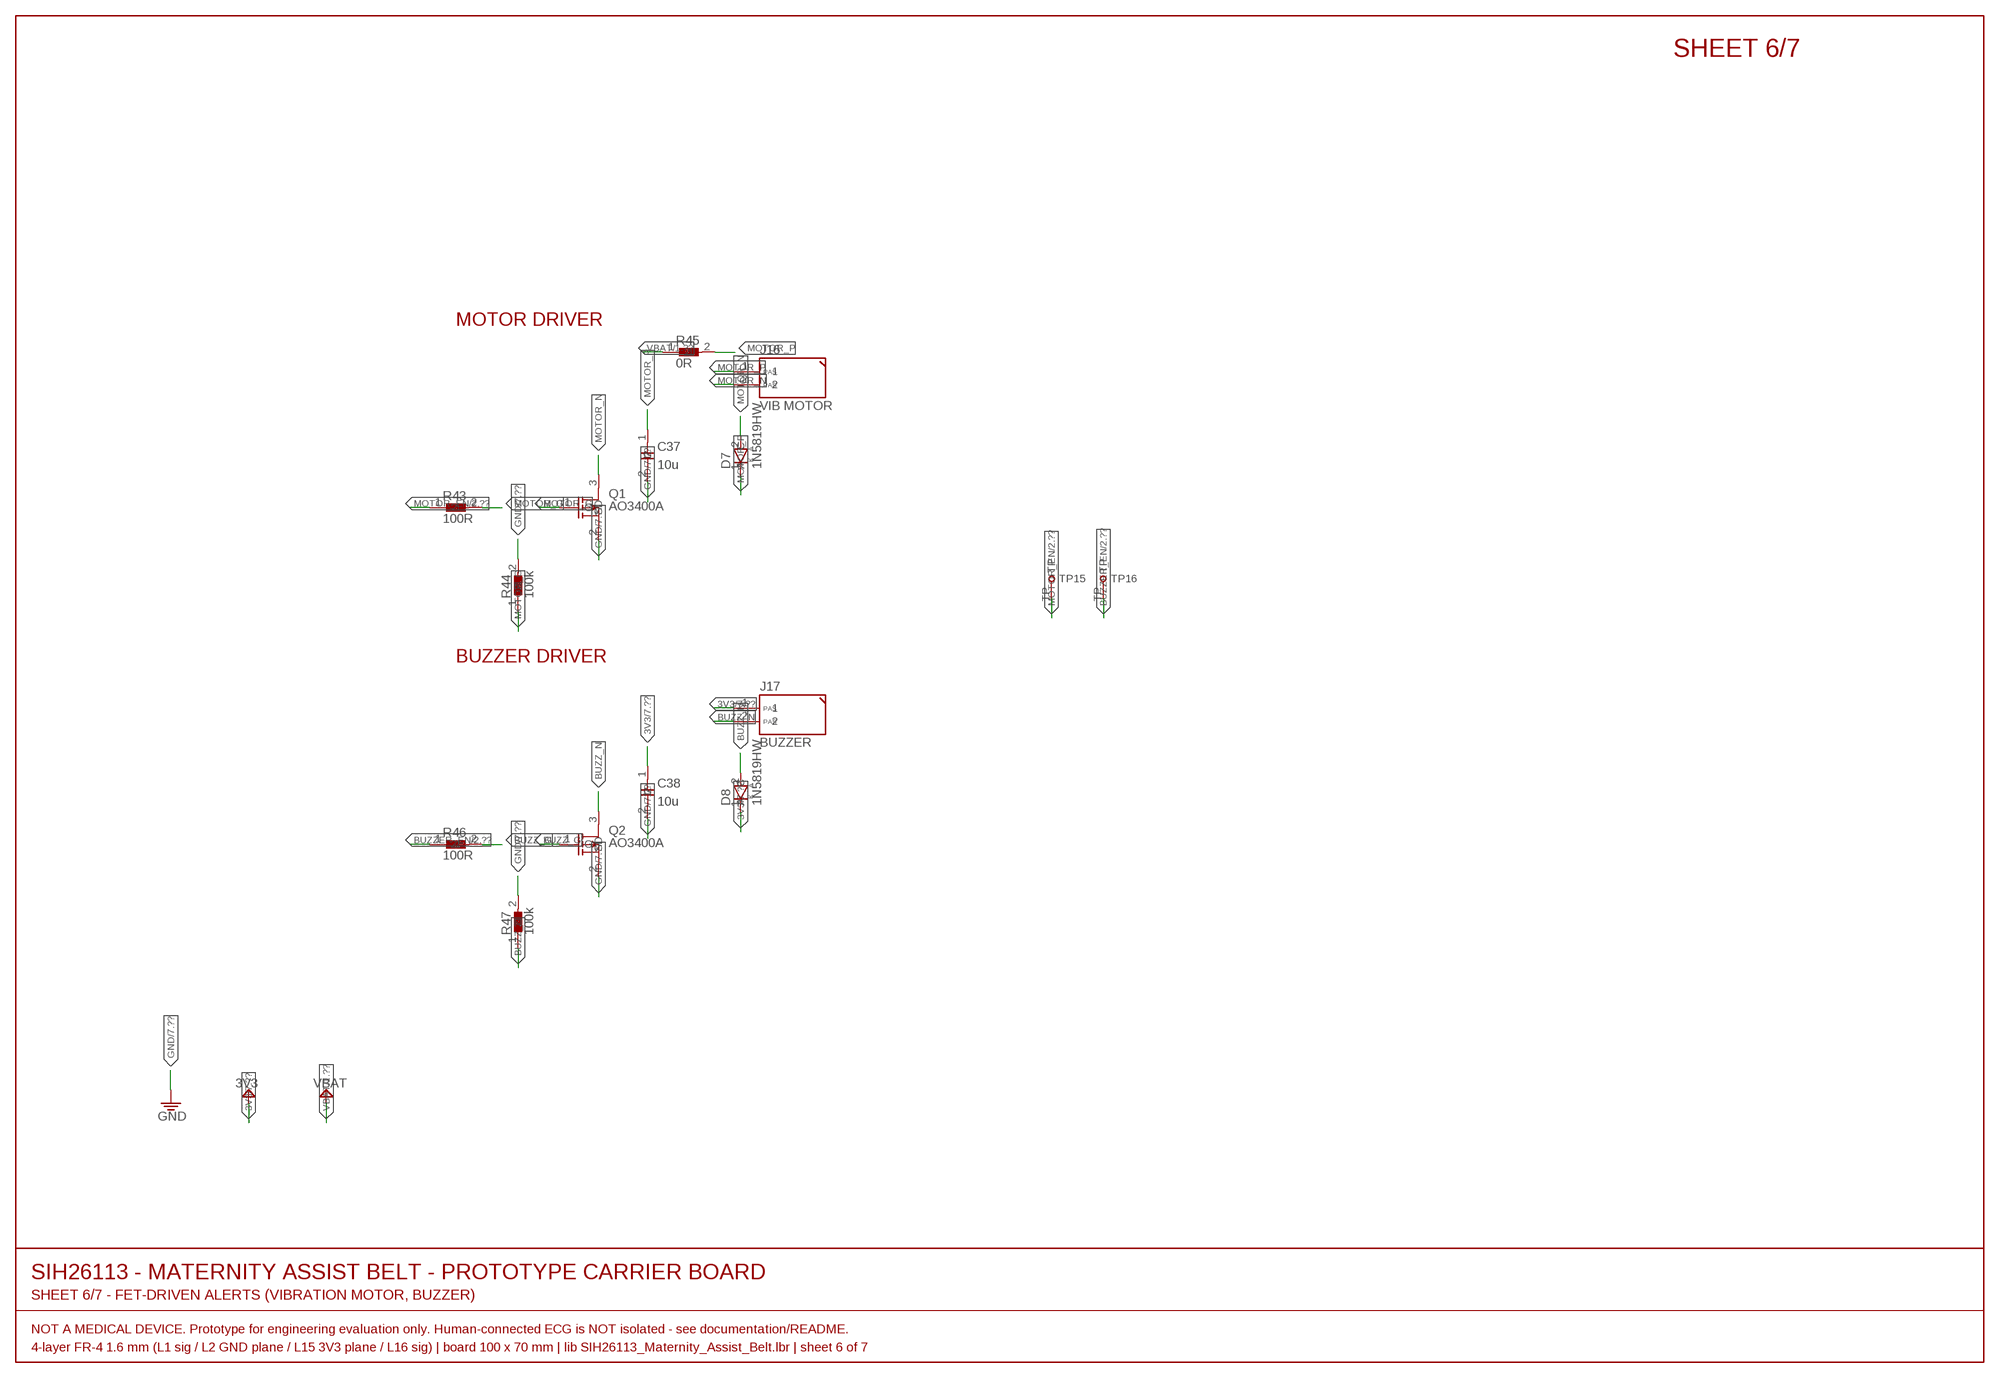
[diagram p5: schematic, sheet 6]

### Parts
C37  10u  C-0805  [C0805]
C38  10u  C-0805  [C0805]
D7  1N5819HW  DIODE-SOD123  [SOD-123]
D8  1N5819HW  DIODE-SOD123  [SOD-123]
J16  VIB MOTOR  HDR-1X2  [HDR-1X2]
J17  BUZZER  HDR-1X2  [HDR-1X2]
Q1  AO3400A  NMOS-SOT23  [SOT-23-3]
Q2  AO3400A  NMOS-SOT23  [SOT-23-3]
R43  100R  R-0805  [R0805]
R44  100k  R-0805  [R0805]
R45  0R  R-0805  [R0805]
R46  100R  R-0805  [R0805]
R47  100k  R-0805  [R0805]
TP15  MOTOR_EN  TESTPOINT  [TESTPOINT-1.5]
TP16  BUZZER_EN  TESTPOINT  [TESTPOINT-1.5]

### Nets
3V3 [power]: C38.1 D8.1(C) J17.1 ; also sheet 1,2,3,4,5,7
BUZZ_G: Q2.1(G) R46.2 R47.1
BUZZ_N: D8.2(A) J17.2 Q2.3(D)
BUZZER_EN: R46.1 TP16.TP ; also sheet 2
GND [power]: C37.2 C38.2 Q1.2(S) Q2.2(S) R44.2 R47.2 ; also sheet 1,2,3,4,5,7
MOTOR_EN: R43.1 TP15.TP ; also sheet 2
MOTOR_G: Q1.1(G) R43.2 R44.1
MOTOR_N [motor]: D7.2(A) J16.2 Q1.3(D)
MOTOR_P [motor]: C37.1 D7.1(C) J16.1 R45.2
VBAT [power]: R45.1 ; also sheet 1

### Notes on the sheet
- SHEET 6/7
- MOTOR DRIVER
- BUZZER DRIVER
- SIH26113 - MATERNITY ASSIST BELT - PROTOTYPE CARRIER BOARD
- SHEET 6/7 - FET-DRIVEN ALERTS (VIBRATION MOTOR, BUZZER)
- NOT A MEDICAL DEVICE. Prototype for engineering evaluation only. Human-connected ECG is NOT isolated - see documentation/README.
- 4-layer FR-4 1.6 mm (L1 sig / L2 GND plane / L15 3V3 plane / L16 sig) | board 100 x 70 mm | lib SIH26113_Maternity_Assist_Belt.lbr | sheet 6 of 7

## Sheet 7 of 7: SHEET 7/7 - USER INPUT AND STORAGE (SOS, microSD)
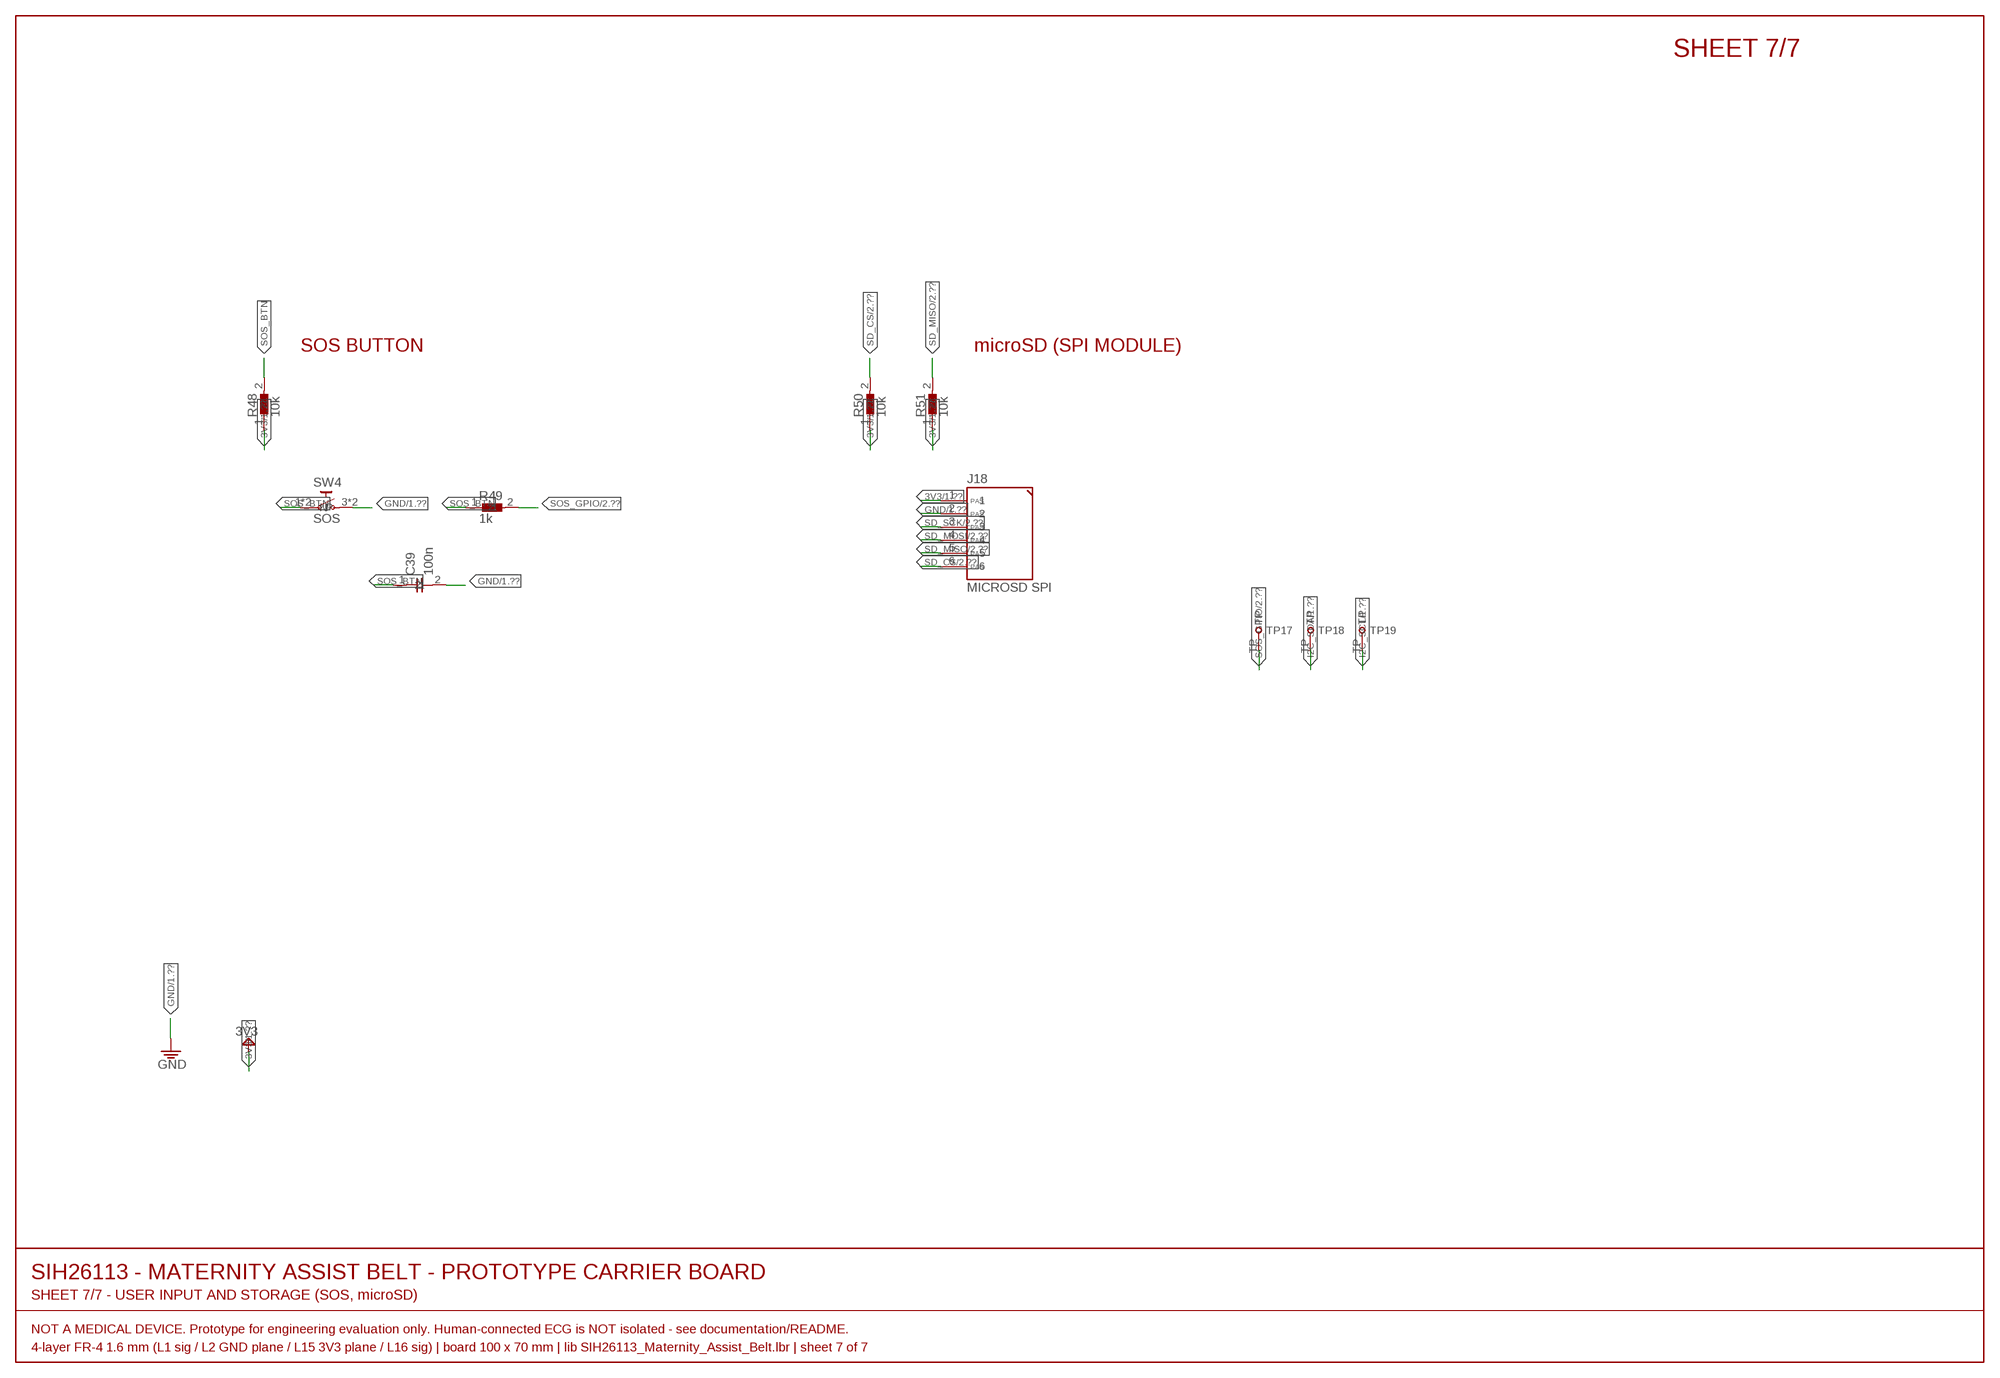
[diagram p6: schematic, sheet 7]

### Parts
C39  100n  C-0805  [C0805]
J18  MICROSD SPI  HDR-1X6  [HDR-1X6]
R48  10k  R-0805  [R0805]
R49  1k  R-0805  [R0805]
R50  10k  R-0805  [R0805]
R51  10k  R-0805  [R0805]
SW4  SOS  SW-TACT-6MM  [TACT-6X6-THT]
TP17  SOS_GPIO  TESTPOINT  [TESTPOINT-1.5]
TP18  I2C_SDA  TESTPOINT  [TESTPOINT-1.5]
TP19  I2C_SCL  TESTPOINT  [TESTPOINT-1.5]

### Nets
3V3 [power]: J18.1 R48.1 R50.1 R51.1 ; also sheet 1,2,3,4,5,6
GND [power]: C39.2 J18.2 SW4.3(N) SW4.4(N) ; also sheet 1,2,3,4,5,6
I2C_SCL: TP19.TP ; also sheet 1,2,3
I2C_SDA: TP18.TP ; also sheet 1,2,3
SD_CS: J18.6 R50.2 ; also sheet 2
SD_MISO: J18.5 R51.2 ; also sheet 2
SD_MOSI: J18.4 ; also sheet 2
SD_SCK: J18.3 ; also sheet 2
SOS_BTN: C39.1 R48.2 R49.1 SW4.1(P) SW4.2(P)
SOS_GPIO: R49.2 TP17.TP ; also sheet 2

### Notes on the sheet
- SHEET 7/7
- SOS BUTTON | microSD (SPI MODULE)
- SIH26113 - MATERNITY ASSIST BELT - PROTOTYPE CARRIER BOARD
- SHEET 7/7 - USER INPUT AND STORAGE (SOS, microSD)
- NOT A MEDICAL DEVICE. Prototype for engineering evaluation only. Human-connected ECG is NOT isolated - see documentation/README.
- 4-layer FR-4 1.6 mm (L1 sig / L2 GND plane / L15 3V3 plane / L16 sig) | board 100 x 70 mm | lib SIH26113_Maternity_Assist_Belt.lbr | sheet 7 of 7

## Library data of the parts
C1-C8 C10-C39 = SIH26113_Maternity_Assist_Belt:C-0805: Chip capacitor, 0805 (2012 metric)
D1-D4 = SIH26113_Maternity_Assist_Belt:LED-0805: Chip LED, 0805. Pad 1 = cathode.
D5-D8 = SIH26113_Maternity_Assist_Belt:DIODE-SOD123: Schottky/rectifier diode, SOD-123. Pad 1 = cathode (band).
H1-H4 = SIH26113_Maternity_Assist_Belt:MOUNTHOLE-M2: M2 plated mounting hole, GND-stitched
J1 = SIH26113_Maternity_Assist_Belt:JST-PH-2: JST PH 2.00 mm 2-circuit top-entry header (S2B-PH-K-S). Li-Po battery input.
J2 = SIH26113_Maternity_Assist_Belt:HDR-1X4: 1x4 2.54 mm pin header
J3 J9-J14 J16 J17 = SIH26113_Maternity_Assist_Belt:HDR-1X2: 1x2 2.54 mm pin header
J4 J6 = SIH26113_Maternity_Assist_Belt:HDR-1X5: 1x5 2.54 mm pin header
J5 J18 = SIH26113_Maternity_Assist_Belt:HDR-1X6: 1x6 2.54 mm pin header
J7 J15 = SIH26113_Maternity_Assist_Belt:HDR-1X3: 1x3 2.54 mm pin header
J8 = SIH26113_Maternity_Assist_Belt:JST-PH-4: JST PH 2.00 mm 4-circuit top-entry header (S4B-PH-K-S). Load-cell bridge input.
Q1 Q2 = SIH26113_Maternity_Assist_Belt:NMOS-SOT23: N-channel logic-level MOSFET, SOT-23-3. Standard assignment 1 = Gate, 2 = Source, 3 = Drain.
R1-R13 R15-R51 = SIH26113_Maternity_Assist_Belt:R-0805: Chip resistor, 0805 (2012 metric)
SW2-SW4 = SIH26113_Maternity_Assist_Belt:SW-TACT-6MM: 6 x 6 mm through-hole tactile push-button. Leads 1-2 and 3-4 are internally common, so each symbol pin maps to two pads (EAGLE multi-pad connect).
TP1-TP19 = SIH26113_Maternity_Assist_Belt:TESTPOINT: 1.5 mm SMD test point
U1 = SIH26113_Maternity_Assist_Belt:TP4056: NanJing Top Power TP4056-42-SOP8-PP 1 A standalone linear Li-ion charger, 4.2 V float. Pin map from the TP4056 datasheet pin description (page 2).
U2 = SIH26113_Maternity_Assist_Belt:AP2112K-3.3: Diodes AP2112K-3.3TRG1 600 mA CMOS LDO, fixed 3.3 V, with enable. Pin map from AP2112 DS39724 Rev.2-2 pin descriptions (SOT25 column).
U3 = SIH26113_Maternity_Assist_Belt:ESP32-S3-WROOM-1: Espressif ESP32-S3-WROOM-1-N8R2. Xtensa LX7 dual-core, Wi-Fi b/g/n + Bluetooth LE 5, 8 MB flash, 2 MB quad-SPI PSRAM, PCB antenna. Pin map from datasheet v1.8 Table 3-1. IO35/36/37 are free on the -N8R2 (quad PSRAM) variant only.
U4 = SIH26113_Maternity_Assist_Belt:TMP117: TI TMP117AIDRVR high-accuracy digital temperature sensor, WSON-6 (DRV). +/-0.1 C, 1.8-5.5 V, I2C. Pin map from TMP117 SNOSD82D Table 5-1 (WSON column).
U5 = SIH26113_Maternity_Assist_Belt:LSM6DSOX: ST LSM6DSOXTR 6-axis IMU (3-axis accel + 3-axis gyro), LGA-14L. Pin map from LSM6DSOX DS12814 Rev.4 Table 1.
U6 = SIH26113_Maternity_Assist_Belt:AS5600: ams-OSRAM AS5600-ASOM 12-bit contactless magnetic rotary position sensor, SOIC-8. Fixed I2C address 0x36. Pin map from AS5600 DS000365 v1-06 Figure 4.
U7 = SIH26113_Maternity_Assist_Belt:AD8232: Analog Devices AD8232ACPZ-R7 single-lead heart-rate monitor front end. Supply 2.0-3.5 V. Pin map from AD8232 Rev.A Table 3.
U8 = SIH26113_Maternity_Assist_Belt:HX711: Avia Semiconductor HX711 24-bit ADC for bridge sensors, SOP-16L. Pin map from the HX711 English datasheet Table 1.

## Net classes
0 default: width 0.2 mm, drill 0.3 mm, clearance 0.15 mm
1 power: width 0.5 mm, drill 0.4 mm, clearance 0.2 mm
2 motor: width 0.5 mm, drill 0.4 mm, clearance 0.2 mm
3 analog_ecg: width 0.2 mm, drill 0.3 mm, clearance 0.2 mm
